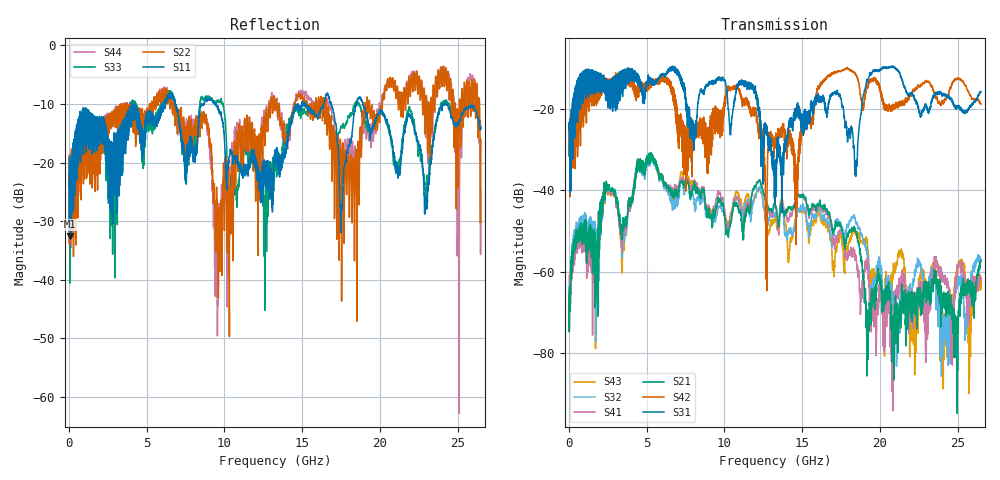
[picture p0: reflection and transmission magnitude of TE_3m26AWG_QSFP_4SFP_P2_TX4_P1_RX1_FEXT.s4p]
!Agilent Technologies,N5222A,MY51421691,A.10.00.00
!Agilent N5222A: A.10.00.00
!Date: Friday, January 30, 2015 12:36:34
!Correction: S11(Full 4 Port(1,2,3,4))
!S12(Full 4 Port(1,2,3,4))
!S13(Full 4 Port(1,2,3,4))
!S14(Full 4 Port(1,2,3,4))
!S21(Full 4 Port(1,2,3,4))
!S22(Full 4 Port(1,2,3,4))
!S23(Full 4 Port(1,2,3,4))
!S24(Full 4 Port(1,2,3,4))
!S31(Full 4 Port(1,2,3,4))
!S32(Full 4 Port(1,2,3,4))
!S33(Full 4 Port(1,2,3,4))
!S34(Full 4 Port(1,2,3,4))
!S41(Full 4 Port(1,2,3,4))
!S42(Full 4 Port(1,2,3,4))
!S43(Full 4 Port(1,2,3,4))
!S44(Full 4 Port(1,2,3,4))
!S4P File: Measurements: <S11,S12,S13,S14>,
!<S21,S22,S23,S24>,
!<S31,S32,S33,S34>,
!<S41,S42,S43,S44>:
# Hz S  dB  R 50.0
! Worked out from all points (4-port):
!   2650 points, 10 MHz to 26.5 GHz, reference 50 ohm
!   strongest paths, dB at 10 MHz, 6.63 GHz, 13.26 GHz, 19.88 GHz, 26.5 GHz:
!     S31: -25.0, -10.5, -43.3, -10.4, -15.7
!     S42: -24.9, -16.2, -29.7, -13.4, -18.8
!     S21: -64.1, -40.7, -43.5, -61.7, -57.3
!     S41: -69.3, -40.1, -44.0, -70.7, -61.8
!     S32: -61.0, -43.2, -45.6, -57.9, -57.6
!     S43: -68.0, -42.8, -46.7, -61.7, -63.9
!   lowest |S11| = -32.5 dB at 70 MHz (marker M1), VSWR 1.05, Z = 52.4 + j0.257 ohm
!   |S11| at or under -10 dB: start of sweep to 4.075 GHz; 9.453 GHz to 14.73 GHz (5.275 GHz wide, 43.6 % of centre); 18.91 GHz to 24.14 GHz (5.228 GHz wide, 24.3 % of centre)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
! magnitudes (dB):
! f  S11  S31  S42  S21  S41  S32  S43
! 10 MHz  -19.2  -25.0  -24.9  -64.1  -69.3  -61.0  -68.0
! 70 MHz  -32.5  -40.7  -41.6  -66.0  -67.3  -62.4  -66.6
! 5.29 GHz  -12.2  -12.6  -12.6  -32.6  -32.7  -33.0  -33.1
! 9.49 GHz  -10.2  -13.2  -19.9  -44.1  -42.4  -46.1  -44.4
! 12.68 GHz  -24.2  -26.1  -45.6  -43.3  -42.9  -47.6  -48.1
! 19.25 GHz  -13.2  -12.8  -14.1  -73.1  -61.6  -58.6  -56.4
! 26.5 GHz  -14.2  -15.7  -18.8  -57.3  -61.8  -57.6  -63.9
